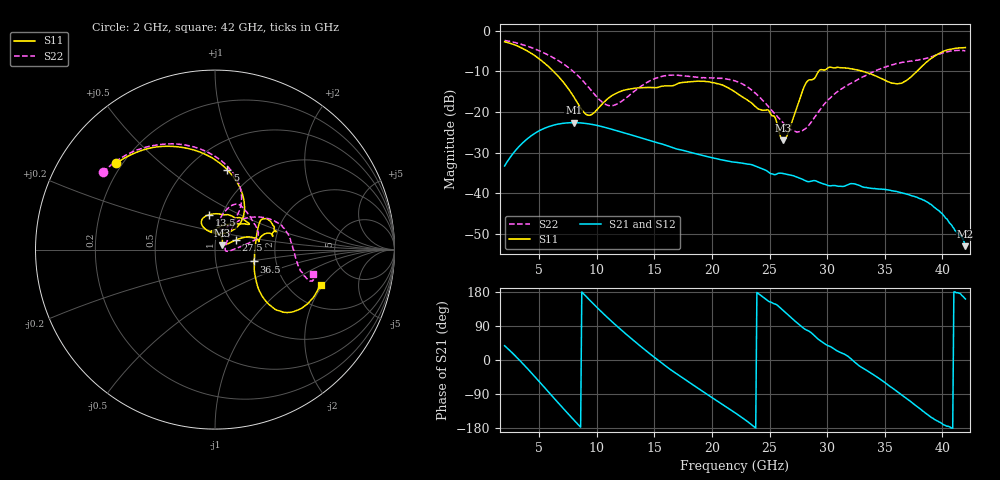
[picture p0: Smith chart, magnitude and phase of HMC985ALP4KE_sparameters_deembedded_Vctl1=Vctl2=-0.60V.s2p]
!s2p File: Measurements: S11, S21, S12, S22
# GHz S dB R 50.0
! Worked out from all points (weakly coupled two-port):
!   401 points, 2 GHz to 42 GHz, reference 50 ohm
!   highest |S21| = -22.64 dB at 8 GHz (marker M1); lowest = -53.0 dB at 42 GHz (marker M2)
!   lowest |S11| = -27.0 dB at 26.2 GHz (marker M3), VSWR 1.09, Z = 53.9 + j2.58 ohm
!   |S11| at or under -10 dB: 6.244 GHz to 29.26 GHz (23.02 GHz wide, 130 % of centre); 33.08 GHz to 37.79 GHz (4.714 GHz wide, 13.3 % of centre)
!   |S22| runs from -25.0 to -2.4 dB; largest |S21 - S12| = 0.00018
!   S11 on the Smith chart (normalised r, x): 2 GHz: 0.18, +0.36; 5 GHz: 0.75, +0.83; 13.5 GHz: 0.87, +0.35; 27.5 GHz: 1.26, +0.14; 36.5 GHz: 1.54, -0.21; 42 GHz: 2.96, -1.88
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2  -2.72 138.9  -33.30 37.7  -33.30 37.7  -2.41 145.4
3.4  -4.14 112.2  -28.09 -3.8  -28.09 -3.8  -3.30 123.0
5  -6.93 81.3  -24.64 -56.7  -24.65 -56.7  -4.93 98.4
8  -16.27 46.7  -22.64 -157.9  -22.64 -157.9  -10.13 61.6
8.7  -19.46 59.0  -22.73 179.5  -22.73 179.5  -12.06 57.7
9.5  -20.73 91.1  -23.03 154.5  -23.03 154.5  -14.63 57.2
11.1  -16.42 118.0  -24.11 107.2  -24.11 107.2  -18.45 73.4
13.5  -14.11 100.1  -26.10 43.7  -26.10 43.7  -14.38 79.0
15.4  -13.88 74.0  -27.70 -2.0  -27.70 -2.0  -11.44 68.3
18.9  -12.45 37.6  -30.51 -76.8  -30.51 -76.8  -11.51 40.6
22  -15.07 53.9  -32.38 -139.1  -32.38 -139.1  -12.36 15.3
24.9  -19.57 95.6  -34.80 155.2  -34.81 155.2  -18.67 2.9
26.2  -27.00 32.3  -35.19 129.9  -35.20 129.9  -22.73 -7.3
27.5  -17.86 24.4  -36.19 95.0  -36.19 95.1  -24.90 2.4
28.1  -13.21 18.3  -36.91 80.8  -36.95 81.1  -24.16 18.4
28.7  -12.06 10.9  -36.97 69.7  -36.95 69.9  -22.17 32.5
31  -9.04 21.6  -38.31 21.9  -38.32 22.2  -14.78 52.2
33.3  -10.20 32.8  -38.59 -25.0  -38.60 -25.2  -11.11 40.5
35.4  -12.67 11.4  -39.29 -68.7  -39.25 -68.1  -8.62 25.0
36.5  -12.89 -17.0  -39.94 -92.8  -39.96 -93.0  -7.80 16.0
39.6  -5.79 -42.7  -44.12 -161.1  -44.08 -161.9  -5.89 -15.6
42  -4.15 -18.5  -53.05 161.1  -53.07 161.7  -4.95 -14.2
